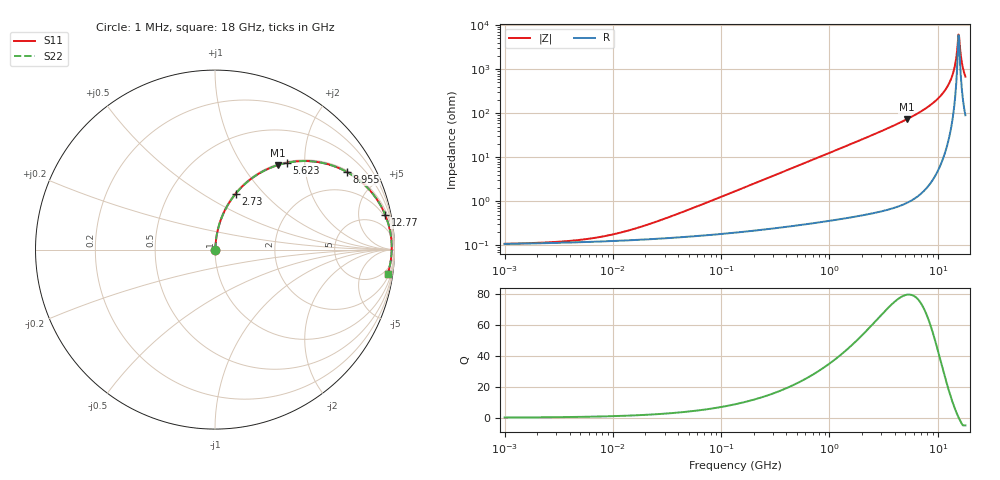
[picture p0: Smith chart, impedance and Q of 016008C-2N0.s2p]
# MHz S MA R 50
!Freq  MagS11  AngS11  MagS21  AngS21  MagS12  AngS12  MagS22  AngS22
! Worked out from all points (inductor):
!   801 points, 1 MHz to 18 GHz, reference 50 ohm
!   read as one part in series: L = 2 nH near 35.74 MHz
!   highest Q = 79.3 at 5.161 GHz (marker M1), where L = 2.25 nH
!   self-resonance near 15.54 GHz
!   S11 on the Smith chart (normalised r, x): 1 MHz: 1.00, +0.00; 2.73 GHz: 1.01, +0.71; 5.623 GHz: 1.02, +1.62; 8.955 GHz: 1.06, +3.35; 12.77 GHz: 1.58, +9.69; 18 GHz: 3, -14
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1  0.001088 6.6  0.9989 -0.0  0.9989 -0.0  0.001088 6.6
5.161289  0.00135 28.6  0.9988 -0.0  0.9988 -0.0  0.00135 28.6
11.30264  0.001907 48.0  0.9987 -0.1  0.9987 -0.1  0.001907 48.0
26.31463  0.003594 66.6  0.9986 -0.2  0.9986 -0.2  0.003594 66.6
134.1641  0.01694 82.4  0.9979 -1.0  0.9979 -1.0  0.01694 82.4
692.4595  0.08664 83.0  0.9931 -5.0  0.9931 -5.0  0.08664 83.0
1426.332  0.1772 78.5  0.9801 -10.2  0.9801 -10.2  0.1772 78.5
2729.811  0.332 69.7  0.938 -19.4  0.938 -19.4  0.332 69.7
3530.478  0.4213 64.3  0.901 -24.9  0.901 -24.9  0.4213 64.3
5160.898  0.5852 53.5  0.8036 -35.8  0.8036 -35.8  0.5852 53.5
5622.881  0.6265 50.5  0.7716 -38.8  0.7716 -38.8  0.6265 50.5
7183.576  0.7482 40.8  0.6532 -48.4  0.6532 -48.4  0.7482 40.8
8955.387  0.8522 30.5  0.508 -58.4  0.508 -58.4  0.8522 30.5
11028.31  0.9313 19.7  0.3367 -68.6  0.3367 -68.6  0.9313 19.7
12774.33  0.968 11.5  0.1995 -75.1  0.1995 -75.1  0.968 11.5
13917.83  0.9801 6.6  0.1157 -76.8  0.1157 -76.8  0.9801 6.6
14438.73  0.9831 4.5  0.0795 -75.5  0.0795 -75.5  0.9831 4.5
14979.11  0.9846 2.4  0.04396 -68.3  0.04396 -68.3  0.9846 2.4
15539.73  0.9847 0.3  0.016 -16.5  0.016 -16.5  0.9847 0.3
16121.32  0.9834 -1.8  0.03602 61.6  0.03602 61.6  0.9834 -1.8
17139.42  0.9781 -5.3  0.09482 74.0  0.09482 74.0  0.9781 -5.3
18000  0.9711 -8.1  0.1426 74.3  0.1426 74.3  0.9711 -8.1
